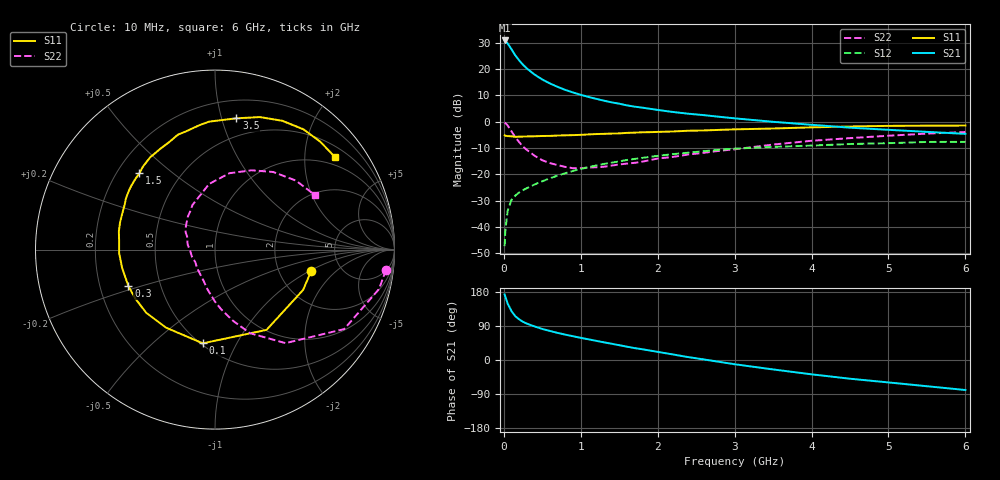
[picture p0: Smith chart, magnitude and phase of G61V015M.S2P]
! SIEMENS Small Signal Semiconductors
! BFG193
! Si NPN RF Bipolar Junction Transistor in SOT223
! VCE = 1 V  IC = 15 mA
! Common Emitter S-Parameters:  August  1996
# GHz  S  MA  R  50
!  f  S11  S21  S12  S22
! GHz  MAG  ANG  MAG  ANG  MAG  ANG  MAG  ANG
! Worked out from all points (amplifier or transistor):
!   36 points, 10 MHz to 6 GHz, reference 50 ohm
!   highest |S21| = 30.9 dB at 10 MHz (marker M1)
!   |S21| within 3 dB of that: start of sweep to 91.45 MHz
!   unconditionally stable (mu >= 1): 697.4 MHz to 2.977 GHz; 3.303 GHz to 3.519 GHz
!   at 250 MHz: K = 0.68, MSG = 23.8 dB, |S12| = -26.0 dB
!   at 1.4 GHz: K = 1.07, MAG = 9.9 dB, |S12| = -15.6 dB
!   at 6 GHz: K = 0.96, MSG = 1.5 dB, |S12| = -7.7 dB
!   S11 on the Smith chart (normalised r, x): 10 MHz: 3.05, -1.04; 100 MHz: 0.51, -0.74; 300 MHz: 0.32, -0.18; 1.5 GHz: 0.29, +0.39; 3.5 GHz: 0.34, +1.12; 6 GHz: 0.76, +2.73
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0.01  0.5493 -12.5  34.96 173.0  0.0043 86.7  0.9593 -6.8
0.02  0.5399 -24.6  34.21 167.1  0.0086 81.0  0.94 -13.5
0.05  0.5315 -57.3  30.68 148.6  0.0204 67.7  0.8451 -31.6
0.1  0.5266 -97.4  23.68 128.9  0.0327 57.0  0.6525 -53.0
0.15  0.5134 -122.1  18.1 115.3  0.0394 51.3  0.5048 -67.3
0.2  0.5203 -137.5  14.58 107.1  0.0453 50.1  0.4082 -75.9
0.25  0.5211 -148.4  12.03 100.7  0.05 49.9  0.3351 -84.0
0.3  0.5236 -157.1  10.23 95.9  0.0545 50.8  0.2899 -90.0
0.4  0.5273 -168.7  7.851 88.5  0.064 51.6  0.2247 -100.9
0.5  0.5345 -178.0  6.331 81.9  0.0736 51.9  0.1846 -110.3
0.6  0.536 175.2  5.32 76.6  0.0841 52.6  0.1632 -119.2
0.7  0.5453 169.2  4.583 71.5  0.0944 52.3  0.1492 -128.6
0.8  0.5504 163.9  4.009 66.9  0.105 51.2  0.1381 -138.4
1.1  0.5721 150.2  2.952 54.5  0.1364 47.9  0.1343 -163.1
1.5  0.5981 134.7  2.196 39.1  0.1758 40.5  0.1537 170.6
1.7  0.6186 128.4  1.929 31.4  0.1958 36.9  0.1651 158.2
2.2  0.6511 113.1  1.527 14.6  0.2417 25.6  0.2139 138.3
2.8  0.6978 97.4  1.238 -4.9  0.2921 12.0  0.2791 116.6
3.5  0.7412 80.7  0.994 -24.9  0.3319 -5.2  0.3674 95.1
4.5  0.8097 62.4  0.769 -49.4  0.3762 -24.4  0.4868 65.2
5.5  0.8398 45.8  0.64 -69.2  0.4117 -46.7  0.5928 40.4
6  0.844 37.9  0.586 -79.2  0.4127 -59.5  0.6354 28.4
